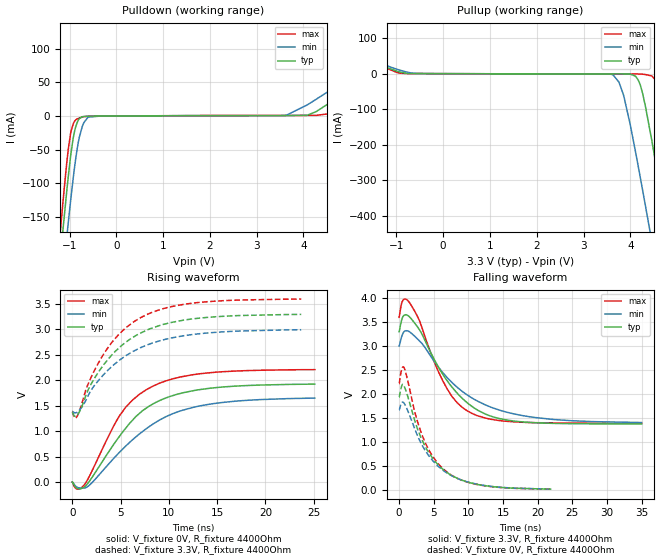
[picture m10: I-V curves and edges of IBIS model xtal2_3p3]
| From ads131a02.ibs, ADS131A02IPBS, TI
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|   xtal2_3p3 Model
[Model]   xtal2_3p3
Model_type   Output
Polarity   Inverting
Vmeas = 1.65
Vref = 0
Cref = 2pF
Rref = 4400
|   typ   min   max
|   (nom PVT)   (fast PVT)   (slow PVT)
C_comp   1.633e-12   1.617e-12   1.642e-12
| Where nom  PVT is Nominal Process, 3.3V, 27C
|   Fast PVT is Strong Process,  3.6V, -40C
|   Slow PVT is Weak Process,   3V, 125C
[Voltage Range]   3.3   3   3.6
|Junction Temperature
[Temperature Range]   27   125   -40
[Pullup Reference]   3.3   3   3.6
[Pulldown Reference]   0   0   0
[Power Clamp Reference]   3.3   3   3.6
[GND Clamp Reference]   0   0   0
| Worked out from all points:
|   slope of the pulldown table from 0 to 0.495 V, typ, clamps not added: 3.06 kohm
|   slope of the pullup table from 0 to 0.495 V, typ, clamps not added: 3.07 kohm
|   falling waveform, V_fixture 3.3V, R_fixture 4400Ohm: 20-80 % time 5.95ns typ, 8.21ns min, 4.47ns max; typ from 3.3 V to 1.38 V
|   rising waveform, V_fixture 0V, R_fixture 4400Ohm: 20-80 % time 5.35ns typ, 6.46ns min, 4.69ns max; typ from 0 V to 1.92 V
|   rising waveform, V_fixture 3.3V, R_fixture 4400Ohm: 20-80 % time 5.37ns typ, 5.8ns min, 4.98ns max; typ from 1.37 V to 3.29 V
|   falling waveform, V_fixture 0V, R_fixture 4400Ohm: 20-80 % time 4.56ns typ, 4.88ns min, 4.21ns max; typ from 1.93 V to 0.014 V
[Pulldown]
|   Voltage   I(typ)   I(min)   I(max)
-3.3V     -1.921A    -1.881A    -1.984A
-1.254V   -255.1mA   -317.7mA   -218.1mA
-1.147V   -174.8mA   -241.5mA   -133.6mA
-1.026V   -90.16mA   -158.7mA   -49.55mA
-978mV    -60.63mA   -127.4mA   -26.65mA
-891.6mV  -22.57mA   -76.13mA   -7.676mA
-813mV    -6.298mA   -39.54mA   -3.641mA
-603mV    -278.1uA   -1.765mA   -386.3uA
3.61V     613.7uA    876.6uA    718.8uA
4.079V    1.074mA    16.43mA    889.2uA
4.58V     20.43mA    38.77mA    3.673mA
6.6V      119.5mA    132.4mA    110.4mA
[Pullup]
|   Voltage   I(typ)   I(min)   I(max)
-3.3V     119.3mA    118.2mA    126.6mA
-914.1mV  4.113mA    9.396mA    1.213mA
3.63V     -616uA     -3.756mA   -824.4uA
3.855V    -658.8uA   -60.41mA   -826.1uA
4.168V    -18.04mA   -260.4mA   -936.7uA
4.321V    -91.27mA   -370.9mA   -2.469mA
4.458V    -187.8mA   -471.8mA   -6.428mA
4.624V    -314mA     -595.7mA   -52.39mA
4.8V      -452.8mA   -729mA     -180.7mA
5.049V    -652.5mA   -918.7mA   -385.7mA
5.142V    -727.8mA   -989.9mA   -464.2mA
6.6V      -1.924A    -2.117A    -1.725A
[Ramp]
R_load = 4400
|   typ   min   max
dV/dt_r   1.15559/5.39069e-09   0.993839/6.55607e-09   1.32502/4.71753e-09
dV/dt_f   1.15527/5.94797e-09   0.95722/8.20943e-09   1.32645/4.47574e-09
[Falling Waveform]
V_fixture = 3.3V
V_fixture_min = 3V
V_fixture_max = 3.6V
R_fixture = 4400Ohm
|   Time   V(typ)   V(min)   V(max)
0s        3.3V       3V         3.6V
533.6ps   3.612V     3.261V     3.952V
1.476ns   3.613V     3.301V     3.912V
2.815ns   3.367V     3.126V     3.567V
4.851ns   2.781V     2.726V     2.747V
6.951ns   2.273V     2.34V      2.102V
10.45ns   1.748V     1.922V     1.599V
13.58ns   1.522V     1.708V     1.465V
19.18ns   1.404V     1.518V     1.403V
35ns      1.375V     1.405V     1.389V
[Rising Waveform]
V_fixture = 0V
V_fixture_min = 0V
V_fixture_max = 0V
R_fixture = 4400Ohm
|   Time   V(typ)   V(min)   V(max)
0s        134.4uV    226.8uV    245.4uV
533.6ps   -125.3mV   -104.8mV   -139.1mV
1.199ns   -103.2mV   -119.8mV   -65.18mV
2.028ns   84.96mV    -15.55mV   211.3mV
4.851ns   886.5mV    576.4mV    1.289V
6.251ns   1.215V     831mV      1.61V
8.351ns   1.531V     1.137V     1.881V
11.11ns   1.733V     1.389V     2.056V
13.91ns   1.831V     1.517V     2.137V
25.11ns   1.92V      1.646V     2.204V
[Rising Waveform]
V_fixture = 3.3V
V_fixture_min = 3V
V_fixture_max = 3.6V
R_fixture = 4400Ohm
|   Time   V(typ)   V(min)   V(max)
0s        1.367V     1.388V     1.382V
278.3ps   1.288V     1.357V     1.255V
500.5ps   1.31V      1.368V     1.288V
1.072ns   1.52V      1.49V      1.591V
1.836ns   1.882V     1.765V     2.006V
3.829ns   2.434V     2.218V     2.671V
5.551ns   2.741V     2.478V     3.026V
7.651ns   2.973V     2.681V     3.278V
13.21ns   3.214V     2.909V     3.523V
23.71ns   3.287V     2.986V     3.587V
[Falling Waveform]
V_fixture = 0V
V_fixture_min = 0V
V_fixture_max = 0V
R_fixture = 4400Ohm
|   Time   V(typ)   V(min)   V(max)
0s        1.933V     1.664V     2.216V
364.4ps   2.166V     1.819V     2.514V
679.9ps   2.175V     1.813V     2.56V
1.16ns    1.988V     1.679V     2.329V
2.286ns   1.43V      1.262V     1.608V
3.369ns   1.021V     916.9mV    1.122V
4.851ns   657.4mV    608mV      695mV
6.951ns   359.2mV    346mV      365.1mV
11.81ns   100.2mV    102.8mV    95.73mV
21.98ns   14.18mV    14.43mV    14.28mV
